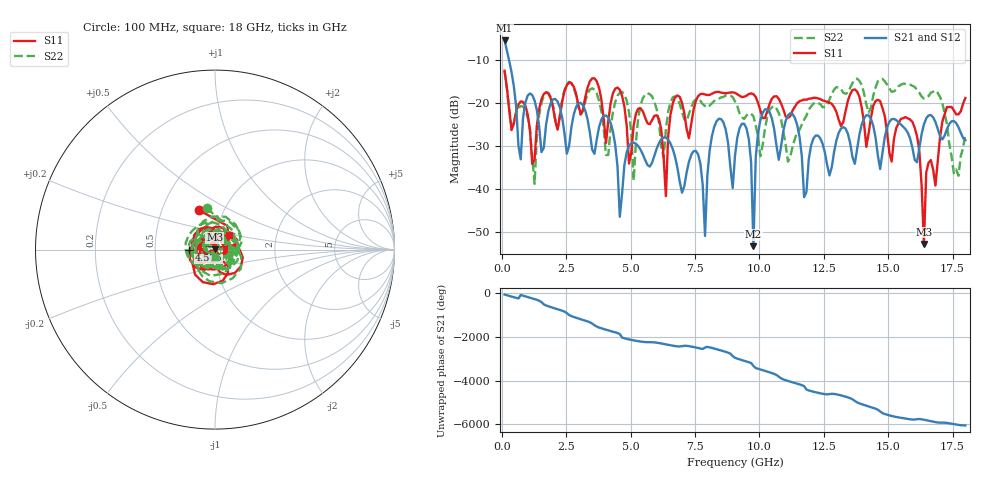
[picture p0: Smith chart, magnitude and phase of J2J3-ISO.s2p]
!Agilent Technologies,E8364B,MY43040528,A.07.50.67
!Agilent E8364B: A.07.50.67
!Date: Wednesday, May 04, 2022 12:36:08
!Correction: S11(Full 2 Port(1,2))
!S21(Full 2 Port(1,2))
!S12(Full 2 Port(1,2))
!S22(Full 2 Port(1,2))
!S2P File: Measurements: S11, S21, S12, S22:
# Hz S  dB  R 50
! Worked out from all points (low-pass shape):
!   201 points, 100 MHz to 18 GHz, reference 50 ohm
!   highest |S21| = -5.43 dB at 100 MHz (marker M1); lowest = -53.4 dB at 9.766 GHz (marker M2)
!   |S21| within 3 dB of the highest: start of sweep to 214.5 MHz
!   lowest |S11| = -52.9 dB at 16.39 GHz (marker M3), VSWR 1.00, Z = 49.8 + j0.127 ohm
!   |S11| at or under -10 dB: start of sweep to end of sweep
!   |S22| runs from -38.9 to -12.6 dB; largest |S21 - S12| = 0.0035
!   S11 on the Smith chart (normalised r, x): 100 MHz: 0.76, +0.36; 4.575 GHz: 0.75, -0.01; 18 GHz: 1.16, +0.19
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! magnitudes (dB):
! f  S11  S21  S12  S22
! 100 MHz  -12.5  -5.4  -5.4  -12.6
! 726.5 MHz  -19.6  -33.2  -33.1  -20.7
! 1.264 GHz  -33.2  -19.4  -19.4  -38.9
! 1.621 GHz  -17.9  -30.5  -30.4  -18.3
! 3.143 GHz  -21.6  -20.5  -20.5  -21.9
! 4.217 GHz  -20.1  -24.7  -24.6  -25.9
! 4.575 GHz  -16.9  -46.6  -46.5  -17.6
! 5.112 GHz  -25.3  -29.2  -29.2  -38.2
! 6.096 GHz  -23.7  -29.4  -29.3  -24.6
! 6.365 GHz  -41.7  -28.1  -28.0  -26.2
! 6.723 GHz  -18.6  -32.6  -32.6  -18.5
! 7.886 GHz  -18.0  -51.0  -51.0  -20.7
! 8.245 GHz  -17.6  -25.6  -25.5  -19.5
! 9.05 GHz  -17.7  -32.3  -32.3  -19.6
! 9.587 GHz  -17.9  -28.5  -28.4  -22.5
! 9.766 GHz  -18.0  -53.4  -53.4  -23.1
! 10.12 GHz  -23.5  -22.3  -22.3  -29.8
! 12.09 GHz  -18.8  -28.3  -28.3  -20.2
! 15.05 GHz  -31.6  -24.4  -24.3  -16.6
! 16.03 GHz  -25.8  -33.3  -33.3  -16.3
! 16.39 GHz  -52.9  -25.0  -25.0  -19.0
! 18 GHz  -18.9  -28.7  -28.6  -27.2
